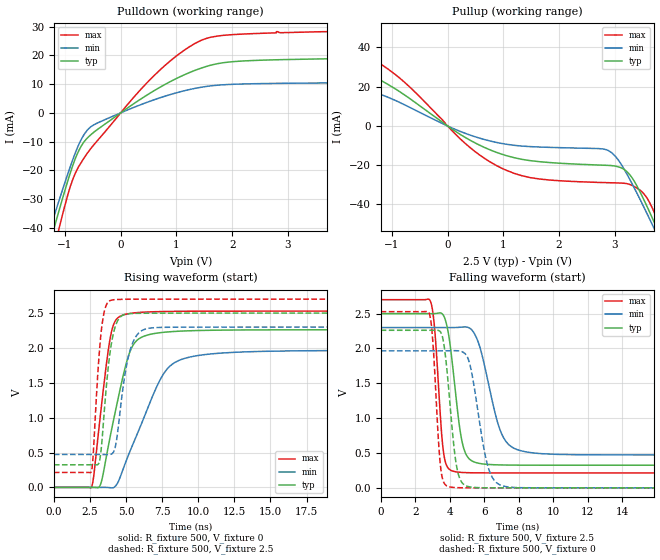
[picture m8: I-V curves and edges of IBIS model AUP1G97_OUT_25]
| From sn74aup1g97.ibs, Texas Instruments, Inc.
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[Model]   AUP1G97_OUT_25
Model_type  Output
Vref =   0
Rref =   1E6
Cref =   30p
Vmeas =   1.25
| variable   typ   min   max
C_comp   2.77pF   1.87pF   4.14pF
| C_pullup   3.12pF   1.87pF   4.14pF
| C_pulldown   2.42pF   2.13pF   2.99pF
[Temperature Range]   40   100   -40
| Ambient temperature   25   85   -40
[Voltage range]   2.5   2.3   2.7
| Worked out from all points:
|   slope of the pulldown table from 0 to 0.375 V, typ, clamps not added: 75.2 ohm
|   slope of the pullup table from 0 to 0.375 V, typ, clamps not added: 55.1 ohm
|   rising waveform, R_fixture 500, V_fixture 0: 20-80 % time 1.41ns typ, 2.4ns min, 866ps max; typ from 0 V to 2.26 V
|   falling waveform, R_fixture 500, V_fixture 2.5: 20-80 % time 627ps typ, 1.07ns min, 401ps max; typ from 2.5 V to 0.325 V
|   rising waveform, R_fixture 500, V_fixture 2.5: 20-80 % time 620ps typ, 793ps min, 473ps max; typ from 0.325 V to 2.5 V
|   falling waveform, R_fixture 500, V_fixture 0: 20-80 % time 522ps typ, 791ps min, 353ps max; typ from 2.26 V to 0 V
[Pulldown]
| AUP1G97_OUT_25
|   Voltage   I(typ)   I(min)   I(max)
-3.6V     -214mA     -193.5mA   -239.7mA
-1.26V    -44.55mA   -39.92mA   -52.42mA
-1.205V   -40.74mA   -36.52mA   -48.02mA
-1.115V   -34.57mA   -31.02mA   -40.91mA
-800mV    -15.22mA   -13.22mA   -20.4mA
-685mV    -10.84mA   -8.445mA   -16.54mA
-540mV    -7.689mA   -4.911mA   -12.5mA
675mV     8.558mA    5.038mA    14.35mA
1.105V    12.9mA     7.5mA      21.28mA
1.52V     16.03mA    9.129mA    25.76mA
2.585V    18.34mA    10.19mA    27.69mA
7.2V      19.61mA    10.73mA    29.61mA
[Pullup]
| AUP1G97_OUT_25
|   Voltage   I(typ)   I(min)   I(max)
-3.6V     37.28mA    23.5mA     50.35mA
-2.355V   24.65mA    15.21mA    35.57mA
-1.425V   26.01mA    17.2mA     35.58mA
-760mV    15.58mA    10.63mA    21.96mA
405mV     -7.279mA   -4.651mA   -11.04mA
1.05V     -15.07mA   -9.293mA   -22.54mA
2.845V    -20.04mA   -12.07mA   -28.88mA
3.17V     -22.17mA   -22.09mA   -29.2mA
3.455V    -33.67mA   -37.48mA   -32.73mA
3.685V    -47.61mA   -50.92mA   -42.5mA
3.82V     -56.28mA   -59.04mA   -51.47mA
7.2V      -294.7mA   -278.7mA   -311.5mA
[Ramp]
| AUP1G97_OUT_25
| variable   typ   min   max
dV/dt_r   1.36/1.41E-09   1.18/2.41E-09   1.52/8.66E-10
dV/dt_f   1.31/6.33E-10   1.10/1.07E-09   1.50/4.11E-10
R_load = 500
[Rising Waveform]
| AUP1G97_OUT_25
R_fixture =   500
C_fixture =   0
L_fixture =   0
V_fixture =   0
V_fixture_min = 0
V_fixture_max = 0
|   Time   V(typ)   V(min)   V(max)
0s        19.04nV    76.96nV    1.464nV
2.625ns   392uV      -8.458uV   11.47mV
3.24ns    46.25mV    442.5uV    1.062V
3.905ns   731mV      -3.995mV   2.141V
4.755ns   1.559V     237.7mV    2.469V
5.285ns   1.953V     523.8mV    2.495V
5.83ns    2.121V     792.7mV    2.508V
7.58ns    2.224V     1.622V     2.522V
9.07ns    2.244V     1.851V     2.526V
32.79ns   2.261V     1.966V     2.528V
[Falling Waveform]
| AUP1G97_OUT_25
R_fixture =   500
C_fixture =   0
L_fixture =   0
V_fixture =   2.5
V_fixture_min = 2.3
V_fixture_max = 2.7
|   Time   V(typ)   V(min)   V(max)
0s        2.5V       2.3V       2.7V
2.89ns    2.5V       2.3V       2.672V
3.135ns   2.5V       2.3V       2.262V
3.635ns   2.476V     2.3V       524.1mV
4.175ns   1.74V      2.3V       240.8mV
5.025ns   447.6mV    2.305V     217.7mV
5.72ns    351mV      2.042V     215.2mV
7ns       328.7mV    782mV      214.5mV
8.13ns    325.7mV    532.1mV    214.4mV
32.79ns   324.7mV    472mV      214.4mV
[Rising Waveform]
| AUP1G97_OUT_25
R_fixture =   500
C_fixture =   0
L_fixture =   0
V_fixture =   2.5
V_fixture_min = 2.3
V_fixture_max = 2.7
|   Time   V(typ)   V(min)   V(max)
0s        324.7mV    472mV      214.4mV
2.6ns     325mV      472mV      227.6mV
2.725ns   324.9mV    472mV      464.8mV
3.1ns     341.2mV    472.1mV    1.796V
3.285ns   558.3mV    471.9mV    2.237V
3.925ns   1.98V      473.9mV    2.681V
4.295ns   2.33V      618.7mV    2.694V
5.255ns   2.491V     1.945V     2.698V
6.355ns   2.498V     2.272V     2.699V
32.79ns   2.5V       2.3V       2.7V
[Falling Waveform]
| AUP1G97_OUT_25
R_fixture =   500
C_fixture =   0
L_fixture =   0
V_fixture =   0
V_fixture_min = 0
V_fixture_max = 0
|   Time   V(typ)   V(min)   V(max)
0s        2.261V     1.966V     2.528V
2.815ns   2.261V     1.966V     2.506V
3.025ns   2.261V     1.966V     2.089V
3.47ns    2.236V     1.966V     302mV
3.93ns    1.449V     1.967V     17.57mV
4.635ns   106.1mV    1.96V      1.734mV
5.19ns    12.68mV    1.75V      350.6uV
6.25ns    813.6uV    280.5mV    30.67uV
7.1ns     173.7uV    26.08mV    6.942uV
32.79ns   -30.53nV   39.65nV    -23.35nV
